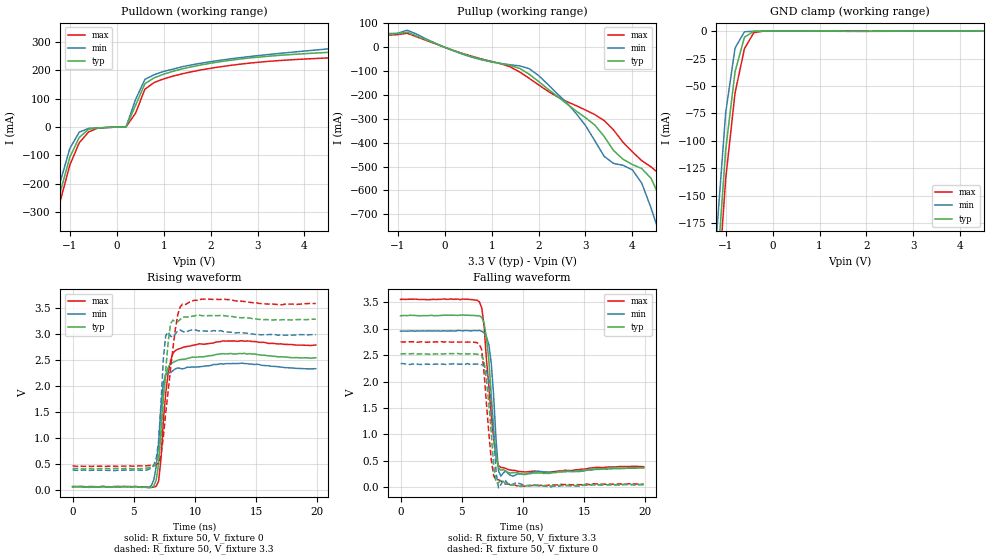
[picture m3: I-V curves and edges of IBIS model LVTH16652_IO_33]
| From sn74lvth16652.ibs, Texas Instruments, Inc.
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|  Model  LVTH16652 IO_33
[Model]   LVTH16652_IO_33
Model_type  I/O
Polarity   Non-Inverting
Enable   Active-Low
Vinl = 0.8V
Vinh = 2.0V
Vmeas = 1.5V
Cref = 50pF
Rref = 500
Vref = 0
| variable   typ   min   max
C_comp   10pf   NA   NA
[Temperature Range]   40   -25   100
| Ambient temperature   25   -40   85
[Voltage range]   3.3   3.0   3.6
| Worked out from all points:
|   slope of the pulldown table from 0 to 0.495 V, typ, clamps not added: 4.39 ohm
|   slope of the pullup table from 0 to 0.495 V, typ, clamps not added: 14.5 ohm
|   GND clamp passes 1 mA (typ) near -0.43 V on its own axis
|   rising waveform, R_fixture 50, V_fixture 0: 20-80 % time 480ps typ, 482ps min, 578ps max; typ from 0.055 V to 2.54 V
|   falling waveform, R_fixture 50, V_fixture 3.3: 20-80 % time 580ps typ, 446ps min, 699ps max; typ from 3.25 V to 0.366 V
|   rising waveform, R_fixture 50, V_fixture 3.3: 20-80 % time 564ps typ, 393ps min, 881ps max; typ from 0.409 V to 3.28 V
|   falling waveform, R_fixture 50, V_fixture 0: 20-80 % time 547ps typ, 456ps min, 579ps max; typ from 2.52 V to 0.048 V
[Pullup]
|   Voltage   I(typ)   I(min)   I(max)
-5V       82.43uA    75.69uA    85.37uA
-2V       71.64uA    63.2uA     76.62uA
-1.8V     71.31uA    62.91uA    50.95mA
-1.6V     53.25mA    56.29mA    50.3mA
-800mV    63.63mA    71.73mA    59mA
2V        -142.9mA   -118mA     -157.2mA
3.4V      -373.7mA   -457.1mA   -307.2mA
4V        -491.2mA   -513.5mA   -438mA
4.6V      -635.2mA   -793.2mA   -534.8mA
4.8V      -738.2mA   -911.8mA   -602mA
5.2V      -951.7mA   -1.149A    -781.6mA
10V       -3.513A    -3.995A    -3.125A
[Pulldown]
|   Voltage   I(typ)   I(min)   I(max)
-5V       -3.744A    -4.018A    -3.358A
-1.4V     -375mA     -352.1mA   -407.6mA
-1.2V     -226.4mA   -190.4mA   -258mA
-1V       -106.1mA   -75.38mA   -133.6mA
-800mV    -36.65mA   -17.86mA   -55.39mA
-400mV    -2.72mA    -3.09mA    -3.446mA
200mV     1.325mA    1.457mA    1.264mA
600mV     152.7mA    167.9mA    133.3mA
1V        186.2mA    196mA      169.6mA
3V        246.1mA    251.4mA    227.9mA
6.8V      294.5mA    355mA      263.6mA
10V       373.2mA    420.9mA    322.3mA
[GND Clamp]
|   Voltage   I(typ)   I(min)   I(max)
-5V       -3.661A    -3.986A    -3.339A
-1.2V     -229.1mA   -189.5mA   -258mA
-1V       -108.3mA   -74.56mA   -134.8mA
-800mV    -37.01mA   -15.45mA   -56.37mA
-600mV    -5.622mA   -650.1uA   -16.06mA
-400mV    -149.5uA   -113.8uA   -1.425mA
-200mV    -48.62uA   -55.97uA   -51.63uA
5V        52.48nA    35.99nA    114.1nA
[Ramp]
| variable   typ   min   max
dV/dt_r   1.566E+00/5.090E-10  1.398E+00/4.750E-10  1.716E+00/6.400E-10
dV/dt_f   1.770E+00/6.130E-10  1.633E+00/4.550E-10  1.944E+00/7.300E-10
R_load = 50
[Rising Waveform]
R_fixture = 50
V_fixture = 0
V_fixture_min = 0
V_fixture_max = 0
C_fixture = 0
L_fixture = 0
|   Time   V(typ)   V(min)   V(max)
0s        55.24mV    66.07mV    63.78mV
6.25ns    40.89mV    49.44mV    51.12mV
6.836ns   194.9mV    456.2mV    71.41mV
7.031ns   498.1mV    887.8mV    170.1mV
7.227ns   1.165V     1.596V     597.7mV
7.422ns   1.843V     2.053V     1.327V
7.617ns   2.211V     2.21V      1.862V
8.008ns   2.427V     2.252V     2.468V
8.594ns   2.488V     2.341V     2.7V
19.88ns   2.537V     2.327V     2.781V
[Falling Waveform]
R_fixture = 50
V_fixture = 3.3
V_fixture_min = 3.0
V_fixture_max = 3.6
C_fixture = 0
L_fixture = 0
|   Time   V(typ)   V(min)   V(max)
0s        3.246V     2.954V     3.555V
6.445ns   3.244V     2.968V     3.51V
6.641ns   3.216V     2.951V     3.397V
6.836ns   3.103V     2.923V     3.042V
7.227ns   2.389V     2.691V     1.896V
7.422ns   1.73V      2.34V      1.354V
7.813ns   595.1mV    888.5mV    577.4mV
8.008ns   360.9mV    314.9mV    410.8mV
8.203ns   323.3mV    209.8mV    373.5mV
19.88ns   366.2mV    367.9mV    388.3mV
[Rising Waveform]
R_fixture = 50
V_fixture = 3.3
V_fixture_min = 3.0
V_fixture_max = 3.6
C_fixture = 0
L_fixture = 0
|   Time   V(typ)   V(min)   V(max)
0s        409.4mV    382.2mV    462mV
6.055ns   417.3mV    381.2mV    463mV
6.641ns   454.4mV    483.4mV    479.6mV
7.031ns   662.1mV    934.3mV    516.5mV
7.422ns   1.772V     2.535V     1.024V
7.617ns   2.312V     2.962V     1.487V
8.008ns   3.19V      2.951V     2.315V
8.594ns   3.229V     3.047V     3.358V
8.984ns   3.315V     3.046V     3.565V
19.88ns   3.276V     2.981V     3.576V
[Falling Waveform]
R_fixture = 50
V_fixture = 0
V_fixture_min = 0
V_fixture_max = 0
C_fixture = 0
L_fixture = 0
|   Time   V(typ)   V(min)   V(max)
0s        2.524V     2.339V     2.753V
6.445ns   2.511V     2.326V     2.708V
6.641ns   2.491V     2.319V     2.598V
6.836ns   2.369V     2.293V     2.156V
7.227ns   1.562V     2.026V     1.004V
7.617ns   396mV      1.001V     218.7mV
7.813ns   85.3mV     286.9mV    137.8mV
8.008ns   81.18mV    -12.05mV   140.1mV
8.398ns   112.3mV    132.8mV    88.5mV
19.88ns   47.61mV    51.12mV    56.15mV
